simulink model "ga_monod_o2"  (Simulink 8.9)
settings: Solver=ode45  StartTime=6.69  StopTime=11.57  MaxStep=0.5  RelTol=1e-6  AbsTol=1e-6  EnableMultiTasking=on
undefined symbols (not defined in the file or in its folder): K, K1, K2, K3, Kga, Muga, Mumax, S0, X0

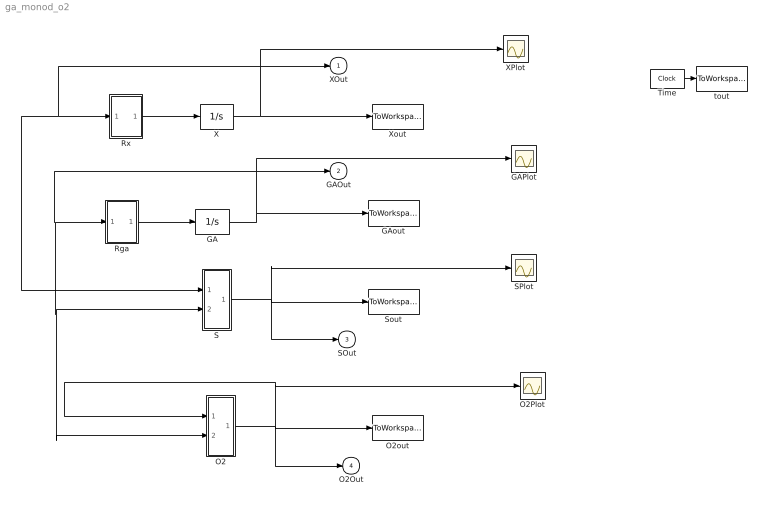
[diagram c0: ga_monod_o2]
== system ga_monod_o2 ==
  GA : Integrator  InitialCondition=X0  UpperSaturationLimit=1000  LowerSaturationLimit=0
  GAPlot : Scope
  GAout : ToWorkspace  VariableName=GAout  SampleTime=-1
  O2 : Subsystem
  O2Plot : Scope
  O2out : ToWorkspace  VariableName=O2out  SampleTime=-1
  Rga : Subsystem
  Rx : Subsystem
  S : Subsystem
  SPlot : Scope
  Sout : ToWorkspace  VariableName=Sout  SampleTime=-1
  Time : Clock
  X : Integrator  InitialCondition=X0  UpperSaturationLimit=1000  LowerSaturationLimit=0
  XPlot : Scope
  Xout : ToWorkspace  VariableName=Xout  SampleTime=-1
  tout : ToWorkspace  VariableName=tout  SampleTime=-1
  XOut : Outport
  GAOut : Outport  Port=2
  SOut : Outport  Port=3
  O2Out : Outport  Port=4
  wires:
  Rga/1(Rga) -> GA/1
  Rx/1(Rx) -> X/1
  Time/1 -> tout/1
  S/1(Sout) -> SPlot/1, SOut/1, Sout/1
  O2/1(O2out) -> O2/1(O2), O2Plot/1, O2Out/1, O2out/1
  X/1 -> Xout/1, XPlot/1, XOut/1, S/1(Rx), Rx/1(X)
  GA/1 -> GAout/1, GAPlot/1, GAOut/1, O2/2(Rga), S/2(Rga), Rga/1(GA)

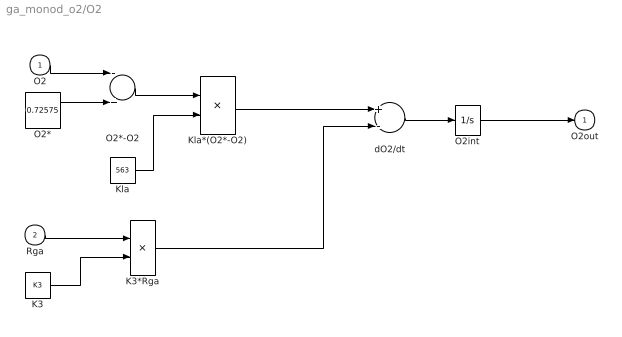
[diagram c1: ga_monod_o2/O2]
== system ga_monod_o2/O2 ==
  O2 : Inport
  Rga : Inport  Port=2
  K3 : Constant  Value=K3
  K3*Rga : Product
  Kla : Constant  Value=563
  Kla*(O2*-O2) : Product
  O2* : Constant  Value=0.72575
  O2*-O2 : Sum  Inputs=-+
  O2int : Integrator  InitialCondition=S0  UpperSaturationLimit=1000  LowerSaturationLimit=0
  dO2/dt : Sum  Inputs=+-
  O2out : Outport
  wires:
  O2int/1 -> O2out/1
  O2/1 -> O2*-O2/1
  K3*Rga/1 -> dO2/dt/2
  dO2/dt/1 -> O2int/1
  O2*/1 -> O2*-O2/2
  Rga/1 -> K3*Rga/1
  K3/1 -> K3*Rga/2
  O2*-O2/1 -> Kla*(O2*-O2)/1
  Kla/1 -> Kla*(O2*-O2)/2
  Kla*(O2*-O2)/1 -> dO2/dt/1

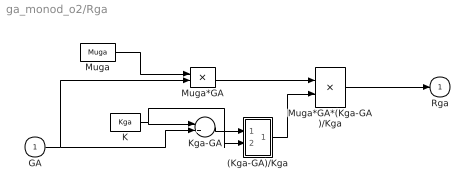
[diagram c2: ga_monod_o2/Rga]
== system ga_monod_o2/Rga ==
  GA : Inport
  (Kga-GA)/Kga : Subsystem
  K : Constant  Value=Kga
  Kga-GA : Sum  Inputs=-+
  Muga : Constant  Value=Muga
  Muga*GA : Product
  Muga*GA*(Kga-GA)/Kga : Product
  Rga : Outport
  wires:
  Muga*GA*(Kga-GA)/Kga/1 -> Rga/1
  Muga/1 -> Muga*GA/1
  Muga*GA/1 -> Muga*GA*(Kga-GA)/Kga/1
  GA/1 -> Kga-GA/2, Muga*GA/2
  K/1 -> (Kga-GA)/Kga/2(Ks+S), Kga-GA/1
  Kga-GA/1 -> (Kga-GA)/Kga/1(Mmax*S)
  (Kga-GA)/Kga/1(out_1) -> Muga*GA*(Kga-GA)/Kga/2

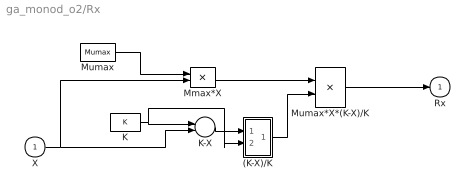
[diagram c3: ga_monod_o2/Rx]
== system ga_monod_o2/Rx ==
  X : Inport
  (K-X)/K : Subsystem
  K : Constant  Value=K
  K-X : Sum  Inputs=+-
  Mmax*X : Product
  Mumax : Constant  Value=Mumax
  Mumax*X*(K-X)/K : Product
  Rx : Outport
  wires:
  Mumax*X*(K-X)/K/1 -> Rx/1
  Mumax/1 -> Mmax*X/1
  Mmax*X/1 -> Mumax*X*(K-X)/K/1
  X/1 -> K-X/2, Mmax*X/2
  K/1 -> (K-X)/K/2(Ks+S), K-X/1
  K-X/1 -> (K-X)/K/1(Mmax*S)
  (K-X)/K/1(out_1) -> Mumax*X*(K-X)/K/2

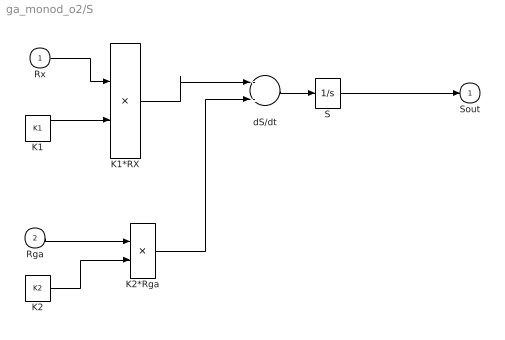
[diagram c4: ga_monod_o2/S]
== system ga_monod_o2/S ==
  Rx : Inport
  Rga : Inport  Port=2
  K1 : Constant  Value=K1
  K1*RX : Product
  K2 : Constant  Value=K2
  K2*Rga : Product
  S : Integrator  InitialCondition=S0  UpperSaturationLimit=1000  LowerSaturationLimit=0
  dS/dt : Sum  Inputs=--
  Sout : Outport
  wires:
  S/1 -> Sout/1
  Rx/1 -> K1*RX/1
  K1*RX/1 -> dS/dt/1
  K2*Rga/1 -> dS/dt/2
  dS/dt/1 -> S/1
  K1/1 -> K1*RX/2
  Rga/1 -> K2*Rga/1
  K2/1 -> K2*Rga/2

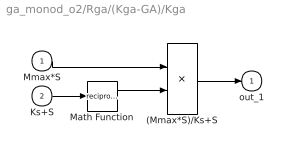
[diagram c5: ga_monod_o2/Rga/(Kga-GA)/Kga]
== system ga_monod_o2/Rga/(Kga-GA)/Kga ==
  Mmax*S : Inport
  Ks+S : Inport  Port=2
  (Mmax*S)/Ks+S : Product
  Math Function : Math  Operator=reciprocal
  out_1 : Outport
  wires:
  Mmax*S/1 -> (Mmax*S)/Ks+S/1
  Ks+S/1 -> Math Function/1
  Math Function/1 -> (Mmax*S)/Ks+S/2
  (Mmax*S)/Ks+S/1 -> out_1/1

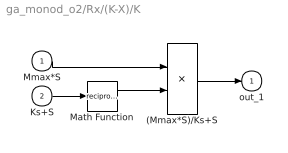
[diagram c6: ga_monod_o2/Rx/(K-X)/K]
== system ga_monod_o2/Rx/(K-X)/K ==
  Mmax*S : Inport
  Ks+S : Inport  Port=2
  (Mmax*S)/Ks+S : Product
  Math Function : Math  Operator=reciprocal
  out_1 : Outport
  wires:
  Mmax*S/1 -> (Mmax*S)/Ks+S/1
  Ks+S/1 -> Math Function/1
  Math Function/1 -> (Mmax*S)/Ks+S/2
  (Mmax*S)/Ks+S/1 -> out_1/1
